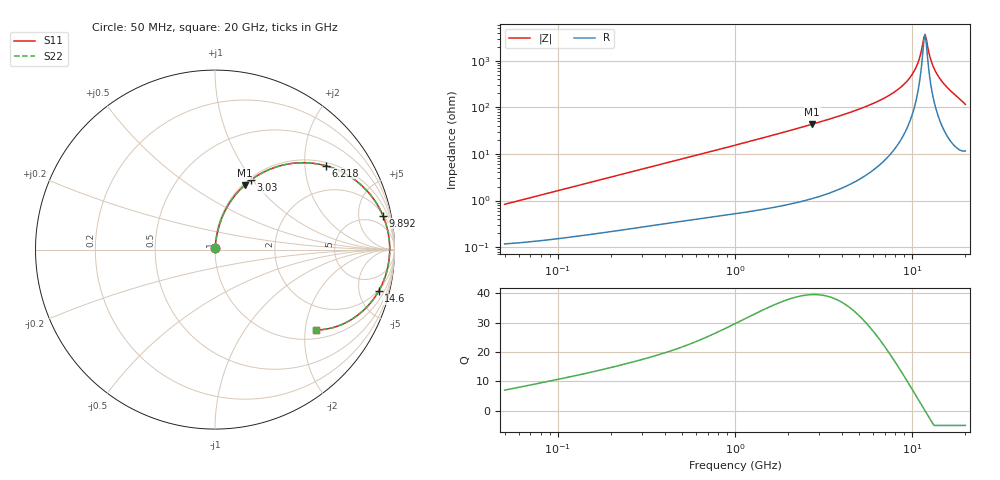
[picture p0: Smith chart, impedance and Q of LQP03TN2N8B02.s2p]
!Murata Part Number: LQP03TN2N8B02
!These Parameters are Measured in Series Mode Connection
!  o--[Z]--o
!Port1  Port2
!  o-------o
!Freq. Start=50[MHz] Stop=20[GHz], 401[Steps]
# Hz S RI R 50
!Freq.(Hz) S11(Real) S11(Imag) S21(Real) S21(Imag) S12(Real) S12(Imag) S22(Real) S22(Imag)
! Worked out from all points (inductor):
!   401 points, 50 MHz to 20 GHz, reference 50 ohm
!   read as one part in series: L = 2.6 nH near 51.52 MHz
!   highest Q = 39.5 at 2.728 GHz (marker M1), where L = 2.53 nH
!   self-resonance near 11.66 GHz
!   S11 on the Smith chart (normalised r, x): 50 MHz: 1.00, +0.02; 3.03 GHz: 1.02, +0.98; 6.218 GHz: 1.10, +2.56; 9.892 GHz: 2.21, +9.45; 14.6 GHz: 1.87, -7.52; 20 GHz: 1.23, -2.30
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5e7  0.00124 0.00819  0.9988 -0.00819  0.9988 -0.00819  0.00124 0.00819
1.364002e8  0.00224 0.0218  0.9978 -0.0218  0.9978 -0.0218  0.00224 0.0218
3.721004e8  0.00636 0.0575  0.9936 -0.0575  0.9936 -0.0575  0.00636 0.0575
1e9  0.0279 0.1486  0.9721 -0.1486  0.9721 -0.1486  0.0279 0.1486
1.766834e9  0.0756 0.2511  0.9244 -0.2511  0.9244 -0.2511  0.0756 0.2511
2.728004e9  0.1649 0.3587  0.8351 -0.3587  0.8351 -0.3587  0.1649 0.3587
3.029571e9  0.1985 0.3864  0.8015 -0.3864  0.8015 -0.3864  0.1985 0.3864
4.34015e9  0.3648 0.4675  0.6352 -0.4675  0.6352 -0.4675  0.3648 0.4675
6.217679e9  0.6162 0.4675  0.3838 -0.4675  0.3838 -0.4675  0.6162 0.4675
7.442007e9  0.7574 0.4038  0.2426 -0.4038  0.2426 -0.4038  0.7574 0.4038
8.774992e9  0.8731 0.2964  0.1269 -0.2964  0.1269 -0.2964  0.8731 0.2964
9.892087e9  0.9355 0.1897  0.0645 -0.1897  0.0645 -0.1897  0.9355 0.1897
1.066139e10  0.9606 0.1134  0.0394 -0.1134  0.0394 -0.1134  0.9606 0.1134
1.098561e10  0.9671 0.0812  0.0329 -0.0812  0.0329 -0.0812  0.9671 0.0812
1.149051e10  0.9727 0.0319  0.0273 -0.0319  0.0273 -0.0319  0.9727 0.0319
1.183995e10  0.9735 -0.00159  0.0265 0.00159  0.0265 0.00159  0.9735 -0.00159
1.220001e10  0.9721 -0.0353  0.0279 0.0353  0.0279 0.0353  0.9721 -0.0353
1.276073e10  0.9653 -0.0859  0.0347 0.0859  0.0347 0.0859  0.9653 -0.0859
1.314879e10  0.9576 -0.1194  0.0424 0.1194  0.0424 0.1194  0.9576 -0.1194
1.460232e10  0.9113 -0.2322  0.0887 0.2322  0.0887 0.2322  0.9113 -0.2322
1.670968e10  0.8058 -0.357  0.1942 0.357  0.1942 0.357  0.8058 -0.357
2e10  0.565 -0.4479  0.435 0.4479  0.435 0.4479  0.565 -0.4479
